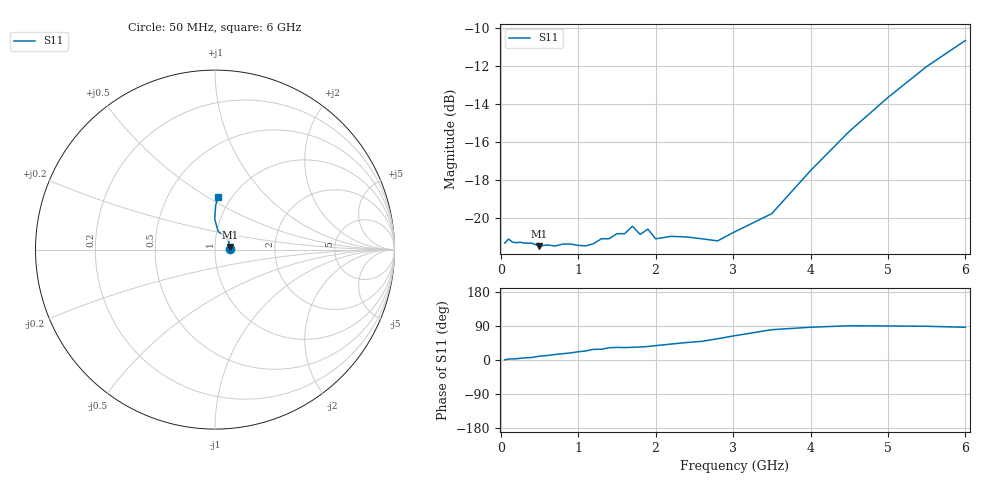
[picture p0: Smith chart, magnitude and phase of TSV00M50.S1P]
! SIEMENS Small Signal Semiconductors
! BAT14-03W
! Si Schottky Diode in SOD323
! IF = 0.5 mA
! S-Parameters:  November  1995
# GHz  S  MA  R  50
!  f  S11
! GHz  MAG  ANG
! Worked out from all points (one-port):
!   34 points, 50 MHz to 6 GHz, reference 50 ohm
!   lowest |S11| = -21.5 dB at 500 MHz (marker M1), VSWR 1.18, Z = 59.1 + j1.76 ohm
!   |S11| at or under -10 dB: start of sweep to end of sweep
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0.05  0.08614 0.4
0.1  0.08831 2.5
0.15  0.08675 2.9
0.4  0.08614 6.7
0.5  0.08458 10.1
0.6  0.08525 11.9
0.7  0.08466 14.5
0.8  0.08564 16.6
1.1  0.08475 24.0
1.2  0.08589 28.2
1.3  0.08847 28.3
1.4  0.08848 32.4
1.5  0.09122 33.2
1.6  0.0912 32.8
1.7  0.09544 33.5
1.8  0.09083 34.2
1.9  0.09374 35.7
2  0.08842 37.9
2.2  0.08977 42.1
2.4  0.08941 46.1
2.6  0.08843 49.4
2.8  0.08732 56.0
3.5  0.103 80.0
4  0.1336 86.4
4.5  0.1693 90.4
5  0.2079 89.8
5.5  0.2508 89.0
6  0.2936 86.3
